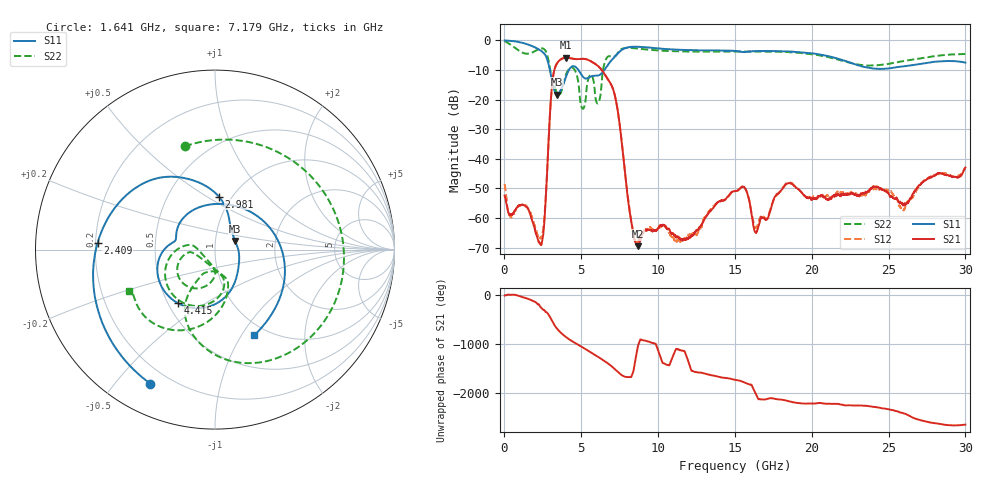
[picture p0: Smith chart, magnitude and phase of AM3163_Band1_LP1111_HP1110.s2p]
!Agilent Technologies,E8364B,MY43040894,A.07.50.67
!Agilent E8364B: A.07.50.67
!Date: Thursday, August 20, 2020 11:59:06
!Correction: S11(Full 2 Port(1,2))
!S21(Full 2 Port(1,2))
!S12(Full 2 Port(1,2))
!S22(Full 2 Port(1,2))
!S2P File: Measurements: S11, S21, S12, S22:
# Hz S  dB  R 50
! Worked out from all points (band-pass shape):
!   3201 points, 10 MHz to 30 GHz, reference 50 ohm
!   highest |S21| = -5.88 dB at 4.021 GHz (marker M1); lowest = -69.5 dB at 8.688 GHz (marker M2)
!   |S21| within 3 dB of the highest: 3.317 GHz to 6.132 GHz (2.815 GHz wide, 59.6 % of centre)
!   lowest |S11| = -18.3 dB at 3.421 GHz (marker M3), VSWR 1.28, Z = 62.2 + j6.04 ohm
!   |S11| at or under -10 dB: 2.959 GHz to 4.198 GHz (1.239 GHz wide, 34.6 % of centre); 4.808 GHz to 6.507 GHz (1.698 GHz wide, 30 % of centre)
!   |S22| runs from -23.1 to -0.3 dB; largest |S21 - S12| = 0.0033
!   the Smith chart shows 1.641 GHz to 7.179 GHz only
!   S11 on the Smith chart (normalised r, x): 1.641 GHz: 0.13, -0.62; 2.409 GHz: 0.21, +0.03; 2.981 GHz: 0.87, +0.57; 4.415 GHz: 0.56, -0.39; 7.179 GHz: 0.86, -1.14
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1e7  -0.07 -4.8  -52.41 -21.1  -48.53 -24.7  -0.34 -11.7
4.973375e8  -0.24 -34.5  -58.99 -2.9  -59.75 -7.1  -1.85 -78.9
9.659312e8  -0.62 -67.2  -55.65 -31.8  -55.82 -32.0  -3.59 -148.9
1.640706e9  -1.63 -115.7  -58.28 -101.0  -57.84 -101.6  -4.45 106.3
2.4092e9  -3.67 176.8  -68.68 83.7  -66.28 -83.6  -2.74 -21.8
2.980884e9  -10.57 85.9  -23.20 -106.1  -23.29 -106.1  -10.23 -120.3
3.421362e9  -18.32 23.2  -7.77 25.4  -7.79 25.4  -17.69 -107.5
4.021162e9  -12.09 -70.6  -5.88 -148.1  -5.90 -147.9  -11.28 -87.6
4.414781e9  -8.80 -124.9  -6.20 128.5  -6.20 128.6  -9.24 -130.9
5.014581e9  -11.67 175.0  -6.29 19.0  -6.27 18.9  -22.52 -159.7
5.979884e9  -11.98 104.8  -8.24 -164.0  -8.25 -164.0  -20.73 -149.6
7.179484e9  -5.59 -65.4  -18.48 -77.1  -18.51 -76.1  -5.45 -154.5
8.688356e9  -2.20 168.8  -69.49 35.1  -67.79 -15.3  -2.80 121.1
1.000979e10  -2.77 100.7  -63.32 -66.0  -63.24 76.2  -3.44 65.7
1.227778e10  -3.36 9.8  -65.70 -117.9  -65.01 88.9  -3.84 -14.9
1.5005e10  -3.59 -74.0  -50.87 66.8  -50.96 67.2  -3.79 -92.5
1.636392e10  -3.64 -104.4  -64.99 138.9  -63.31 11.8  -3.79 -125.7
1.839762e10  -3.74 -154.3  -48.37 -0.5  -48.20 -0.9  -3.98 -177.2
2.000958e10  -4.40 162.7  -53.73 -57.6  -53.22 -51.5  -4.70 135.6
2.274617e10  -7.99 59.9  -52.09 -95.7  -51.76 -92.9  -7.94 20.5
2.500479e10  -9.50 -63.0  -51.64 -171.3  -50.86 -177.5  -7.98 -93.3
3e10  -7.54 105.0  -42.93 -124.9  -43.06 -133.0  -4.64 100.9
